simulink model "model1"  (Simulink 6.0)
settings: Solver=ode45  StartTime=0.0  StopTime=10.0  RelTol=1e-3
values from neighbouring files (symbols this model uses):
  K1 = A2    [fun_F.m]    (also in fun_F6.m = A1; main6.m = 0.5; fun_F7.m; main7.m = 3)
  K2 = A1    [fun_F.m]    (also in fun_F6.m; main6.m = 0.5; fun_F7.m; main7.m = 2)
  K3 = A1    [fun_F.m]    (also in fun_F6.m = A2; main6.m = 0.5; fun_F7.m; main7.m = 0)
libraries: simulink x1

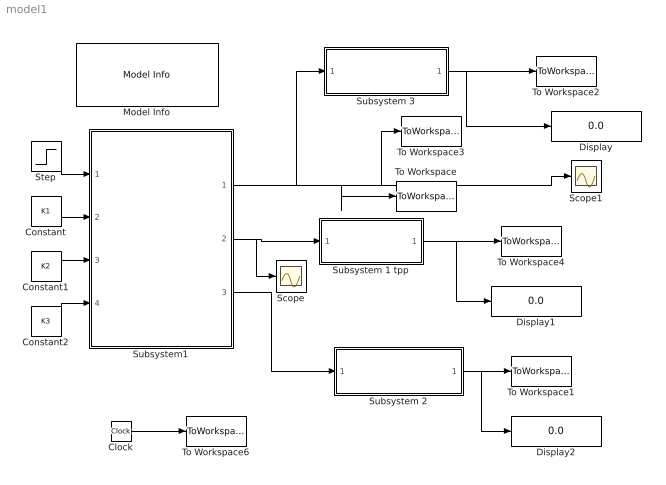
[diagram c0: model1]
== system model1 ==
  Clock : Clock
  Constant : Constant  Value=K1
  Constant1 : Constant  Value=K2
  Constant2 : Constant  Value=K3
  Display : Display
  Display1 : Display
  Display2 : Display
  Model Info : simulink/Model-Wide Utilities/Model Info  InitialBlockCM=None  BlockCM=None  Frame=on  DisplayStringWithTags=|  HorizontalTextAlignment=Center  LeftAlignmentValue=0.5  SourceBlockDiagram=model1  TagMaxNumber=20
      | Model Info
      | 1.Step Time=0(blok Step)
      | 2.In command line input:
      | K1=1,K2=5,K3=1
  Scope : Scope
  Scope1 : Scope
  Step : Step  Time=0  SampleTime=0
  Subsystem 1 tpp : Subsystem
  Subsystem 2 : Subsystem
  Subsystem 3 : Subsystem
  Subsystem1 : Subsystem
  To Workspace : ToWorkspace  VariableName=yout  SampleTime=-1  SaveFormat=Array
  To Workspace1 : ToWorkspace  VariableName=pregsV  SampleTime=-1  SaveFormat=Array
  To Workspace2 : ToWorkspace  VariableName=pregs  SampleTime=-1  SaveFormat=Array
  To Workspace3 : ToWorkspace  VariableName=pregs1  SampleTime=-1  SaveFormat=Array
  To Workspace4 : ToWorkspace  VariableName=tpptek  SampleTime=-1  SaveFormat=Array
  To Workspace6 : ToWorkspace  VariableName=timeout  SampleTime=-1  SaveFormat=Array
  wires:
  Constant2/1 -> Subsystem1/4(In4:K3)
  Constant1/1 -> Subsystem1/3(In3:K2)
  Constant/1 -> Subsystem1/2(In2:K2)
  Step/1 -> Subsystem1/1(In1:input)
  Subsystem1/2(Out2(for tpp)) -> Subsystem 1 tpp/1(In1:Signal), Scope/1
  Subsystem1/1(Out1:for max) -> Scope1/1, To Workspace3/1, To Workspace/1, Subsystem 3/1(In1:Signal)
  Subsystem 3/1(Out1:nepeper.) -> To Workspace2/1, Display/1
  Subsystem 1 tpp/1(Out1:tpp) -> To Workspace4/1, Display1/1
  Subsystem1/3(Out3(for maxV)) -> Subsystem 2/1(In1:Signal)
  Subsystem 2/1(Out1:nepeper.) -> To Workspace1/1, Display2/1
  Clock/1 -> To Workspace6/1

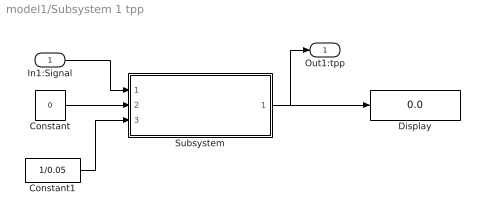
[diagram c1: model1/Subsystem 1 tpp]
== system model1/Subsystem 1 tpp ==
  In1:Signal : Inport  Port=1  LatchInput=off
  Constant : Constant  Value=0
  Constant1 : Constant  Value=1/0.05
  Display : Display
  Subsystem : Subsystem
  Out1:tpp : Outport
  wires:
  In1:Signal/1 -> Subsystem/1(In1:Signal)
  Constant/1 -> Subsystem/2(In2:ustzn)
  Constant1/1 -> Subsystem/3(In3:Lavel)
  Subsystem/1(Out1) -> Display/1, Out1:tpp/1

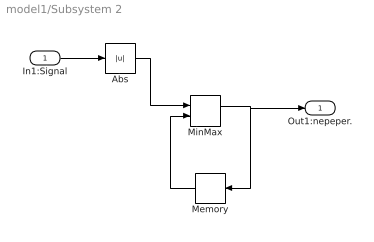
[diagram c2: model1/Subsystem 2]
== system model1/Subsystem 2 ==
  In1:Signal : Inport  Port=1  LatchInput=off
  Abs : Abs
  Memory : Memory  Orientation=left
  MinMax : MinMax  Function=max  Inputs=2
  Out1:nepeper. : Outport
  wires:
  In1:Signal/1 -> Abs/1
  Abs/1 -> MinMax/1
  MinMax/1 -> Out1:nepeper./1, Memory/1
  Memory/1 -> MinMax/2

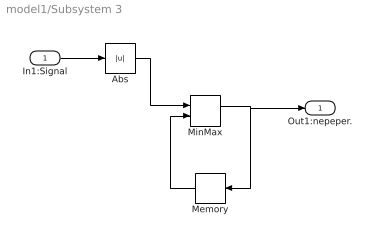
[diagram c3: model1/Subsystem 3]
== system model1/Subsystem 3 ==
  In1:Signal : Inport  Port=1  LatchInput=off
  Abs : Abs
  Memory : Memory  Orientation=left
  MinMax : MinMax  Function=max  Inputs=2
  Out1:nepeper. : Outport
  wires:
  In1:Signal/1 -> Abs/1
  Abs/1 -> MinMax/1
  MinMax/1 -> Out1:nepeper./1, Memory/1
  Memory/1 -> MinMax/2

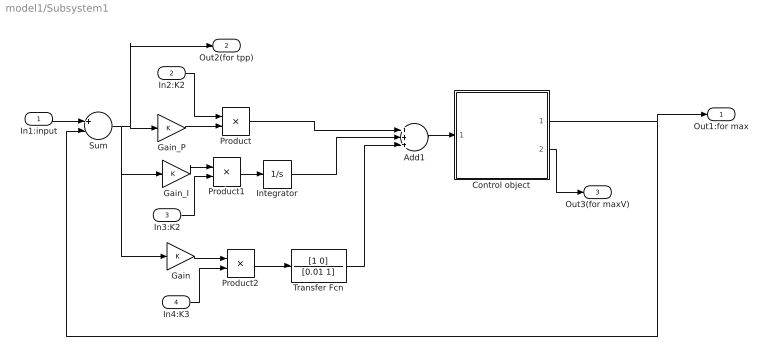
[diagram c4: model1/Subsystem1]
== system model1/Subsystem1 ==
  In1:input : Inport  Port=1  LatchInput=off
  In2:K2 : Inport  Port=2  LatchInput=off
  In3:K2 : Inport  Port=3  LatchInput=off
  In4:K3 : Inport  Port=4  LatchInput=off
  Add1 : Sum  Inputs=+++  OutScaling=2^-10
  Control object : Subsystem
  Gain : Gain
  Gain_I : Gain
  Gain_P : Gain
  Integrator : Integrator
  Product : Product
  Product1 : Product
  Product2 : Product
  Sum : Sum  Inputs=+-  OutScaling=2^-10
  Transfer Fcn : TransferFcn  Numerator=[1 0]  Denominator=[0.01 1]
  Out1:for max : Outport
  Out2(for tpp) : Outport  Port=2
  Out3(for maxV) : Outport  Port=3
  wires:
  Gain_I/1 -> Product1/1
  In3:K2/1 -> Product1/2
  Product1/1 -> Integrator/1
  Gain/1 -> Product2/1
  In4:K3/1 -> Product2/2
  Product2/1 -> Transfer Fcn/1
  Sum/1 -> Gain/1, Gain_I/1, Gain_P/1, Out2(for tpp)/1
  In1:input/1 -> Sum/1
  Integrator/1 -> Add1/2
  Transfer Fcn/1 -> Add1/3
  Add1/1 -> Control object/1(In1)
  Control object/1(Out1) -> Sum/2, Out1:for max/1
  Control object/2(Out2(maxV)) -> Out3(for maxV)/1
  Gain_P/1 -> Product/2
  Product/1 -> Add1/1
  In2:K2/1 -> Product/1

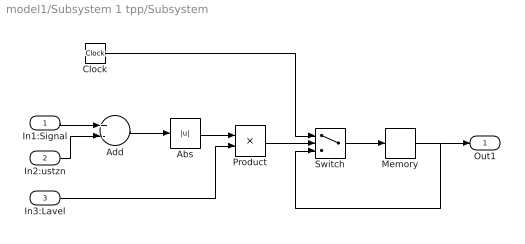
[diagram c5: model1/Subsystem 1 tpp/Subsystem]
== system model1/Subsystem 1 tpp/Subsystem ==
  In1:Signal : Inport  Port=1  LatchInput=off
  In2:ustzn : Inport  Port=2  LatchInput=off
  In3:Lavel : Inport  Port=3  LatchInput=off
  Abs : Abs
  Add : Sum  Inputs=+-  OutScaling=2^-10
  Clock : Clock
  Memory : Memory
  Product : Product
  Switch : Switch  Threshold=1
  Out1 : Outport
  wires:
  In1:Signal/1 -> Add/1
  In2:ustzn/1 -> Add/2
  Add/1 -> Abs/1
  Abs/1 -> Product/1
  In3:Lavel/1 -> Product/2
  Product/1 -> Switch/2
  Clock/1 -> Switch/1
  Switch/1 -> Memory/1
  Memory/1 -> Out1/1, Switch/3

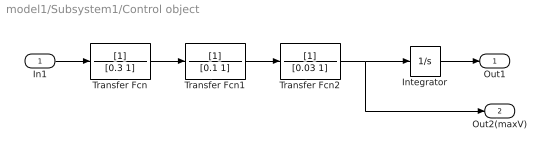
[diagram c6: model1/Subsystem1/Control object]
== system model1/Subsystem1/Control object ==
  In1 : Inport  Port=1  LatchInput=off
  Integrator : Integrator
  Transfer Fcn : TransferFcn  Denominator=[0.3 1]
  Transfer Fcn1 : TransferFcn  Denominator=[0.1 1]
  Transfer Fcn2 : TransferFcn  Denominator=[0.03 1]
  Out1 : Outport
  Out2(maxV) : Outport  Port=2
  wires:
  In1/1 -> Transfer Fcn/1
  Transfer Fcn/1 -> Transfer Fcn1/1
  Transfer Fcn1/1 -> Transfer Fcn2/1
  Transfer Fcn2/1 -> Integrator/1, Out2(maxV)/1
  Integrator/1 -> Out1/1
